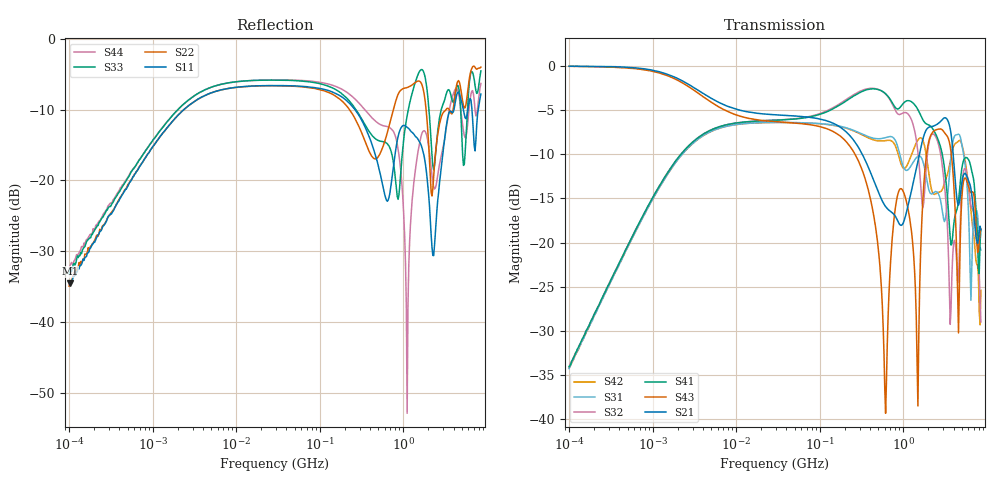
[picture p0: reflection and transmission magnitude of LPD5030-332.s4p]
# MHz S MA R 50
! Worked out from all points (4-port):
!   498 points, 100 kHz to 8.5 GHz, reference 50 ohm
!   strongest paths, dB at 100 kHz, 1.698 MHz, 29.49 MHz, 500.7 MHz, 8.5 GHz:
!     S21: -0.1, -1.2, -5.6, -14.2, -18.6
!     S43: -0.1, -1.3, -6.3, -20.5, -18.5
!     S41: -34.0, -11.4, -6.2, -2.7, -18.5
!     S32: -34.0, -11.4, -6.2, -2.7, -29.0
!     S31: -34.3, -11.5, -6.4, -8.3, -20.8
!     S42: -34.2, -11.6, -6.4, -8.5, -25.4
!   lowest |S11| = -34.5 dB at 102.3 kHz (marker M1), VSWR 1.04, Z = 50.1 + j1.88 ohm
!   |S11| at or under -10 dB: 263.7 MHz to 4.046 GHz (3.782 GHz wide, 176 % of centre); 5.237 GHz to 5.944 GHz (707.6 MHz wide, 12.7 % of centre); 6.642 GHz to 7.91 GHz (1.269 GHz wide, 17.4 % of centre)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
0.1  0.01949 84.7  0.9929 -1.1  0.01935 -92.5  0.01988 87.4
     0.9929 -1.1  0.01792 84.0  0.01989 87.0  0.01949 -92.4
     0.01935 -92.5  0.01989 87.0  0.02182 80.9  0.9916 -1.4
     0.01988 87.4  0.01949 -92.4  0.9916 -1.4  0.02369 88.0
0.1023101  0.0188 85.4  0.9934 -1.2  0.01999 -92.0  0.02012 86.7
           0.9934 -1.2  0.0191 86.3  0.02044 87.1  0.01984 -92.6
           0.01999 -92.0  0.02044 87.1  0.02322 84.3  0.9916 -1.4
           0.02012 86.7  0.01984 -92.6  0.9916 -1.4  0.02504 85.3
90.29583  0.4495 -25.7  0.5044 -31.2  0.4719 144.6  0.523 -2.4
          0.5044 -31.2  0.4433 -24.3  0.5272 -3.1  0.4709 145.3
          0.4719 144.6  0.5272 -3.1  0.4875 -24.0  0.4574 -32.6
          0.523 -2.4  0.4709 145.3  0.4574 -32.6  0.4964 -24.6
614.9063  0.07546 -102.9  0.1597 -149.5  0.3923 -15.9  0.6939 -96.3
          0.1597 -149.5  0.1969 -47.6  0.691 -106.3  0.3771 -12.7
          0.3923 -15.9  0.691 -106.3  0.1848 -90.2  0.01083 -86.2
          0.6939 -96.3  0.3771 -12.7  0.01083 -86.2  0.2413 -129.9
1113.489  0.2365 -166.7  0.1539 -15.5  0.2561 -115.4  0.6336 -164.8
          0.1539 -15.5  0.4517 -141.7  0.5381 174.6  0.2738 -102.5
          0.2561 -115.4  0.5381 174.6  0.2865 -90.8  0.1637 -154.7
          0.6336 -164.8  0.2738 -102.5  0.1637 -154.7  0.002274 -12.4
7080.634  0.1738 120.8  0.1373 55.9  0.1439 167.0  0.213 120.5
          0.1373 55.9  0.6391 -169.9  0.1379 141.4  0.1037 103.8
          0.1439 167.0  0.1379 141.4  0.514 -175.1  0.1802 110.3
          0.213 120.5  0.1037 103.8  0.1802 110.3  0.3648 -165.4
8500  0.4068 -41.6  0.1182 64.5  0.09078 -20.4  0.1184 -20.3
      0.1182 64.5  0.6296 -29.2  0.03559 -47.0  0.05363 -10.0
      0.09078 -20.4  0.03559 -47.0  0.5914 -21.1  0.1191 73.5
      0.1184 -20.3  0.05363 -10.0  0.1191 73.5  0.4827 -36.9
